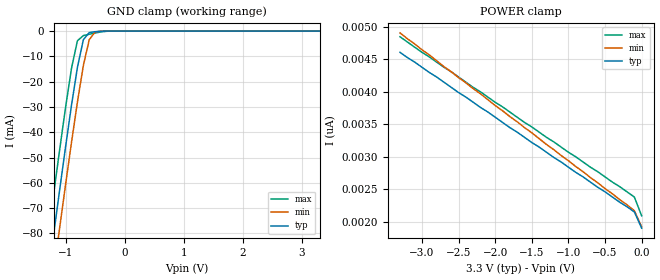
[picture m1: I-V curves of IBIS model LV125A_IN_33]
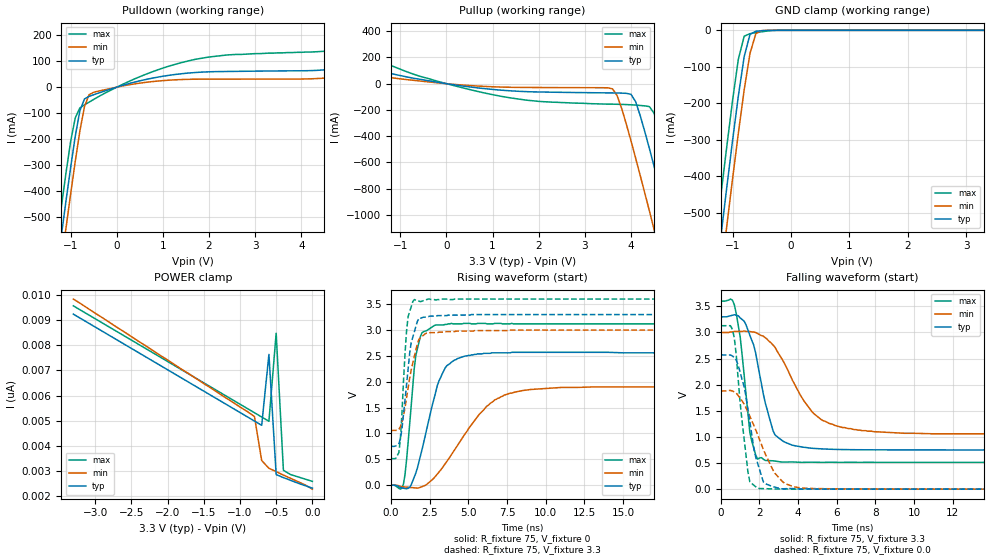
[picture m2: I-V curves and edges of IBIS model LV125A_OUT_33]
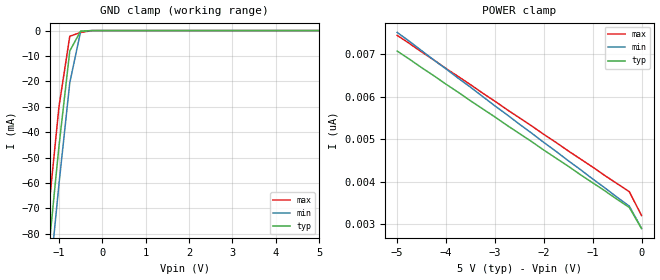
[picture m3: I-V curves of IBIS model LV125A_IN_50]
| TEXAS INSTRUMENTS INCORPORATED
| Standard Linear and Logic Group
| IBIS Model of SN74LV125A
| QUADRUPLE BUS BUFFER GATE WITH 3-STATE OUTPUTS
| SOIC 14-pin (D), SOP 14-pin (NS), SSOP 14-pin (DB), TSSOP 14-pin (PW)
| and TVSOP 14-pin (DGV) Package
[IBIS Ver]   3.2
[Comment Char]  |_char
[File Name]   lv125a.ibs
[File Rev]   2.0 H_die
[Date]   May 26, 2000
[Source]   Data created from HSPICE simulations at TI-SLL.
[Notes]   The following is an IBIS list for the LV125A.
|   Please contact sllibis@ti.com with questions and
|   comments concerning SLL IBIS models.
|   The warning about non-monotonic V-I curves might be reported,
|   but it is nano ampere region and negligible.
[Disclaimer] Property of Texas Instruments Incorporated.  Unauthorized
   reproduction and/or distribution is strictly prohibited.
   This product is protected under copyright law.
   Created 2000, (C) Copyright 2000, Texas Instruments Inc.,
   All Rights Reserved.
   UNLESS THERE IS A SIGNED, WRITTEN AGREEMENT TO THE
   CONTRARY, TEXAS INSTRUMENTS () IS PROVIDING THE IBIS
   MODELS  AND WITHOUT ANY WARRANTY, EXPRESSED OR
   IMPLIED.  TI assumes no liability for:
   1) the accuracy of the IBIS models provided to your
   company;
   2) the proper functioning of these IBIS Models in your
   design or for any resulting applications; or
   3) infringement of patents, copyrights or intellectual
   property rights resulting from your use of these IBIS
   models.
   TI provides IBIS Models as a service to our customers.
   You and your company shall not distribute, sell or give
   these models to anyone else without prior written
   permission from TI.
   TI reserves the right to make changes to our products or
   to discontinue any semiconductor product or service
   without notice, and advises our customers to obtain the
   latest version of relevant information to verify, before
   placing orders, that the information being relied on is
   current.
   Please be aware that your receipt and use of the IBIS
   information provided shall serve as acceptance of these
   terms and conditions.  If you do not accept these terms,
   you should return or destroy the IBIS models and any
   other accompanying information immediately.
|   Component LV125A_D
[Component]   LV125A_D
[Manufacturer]  Texas Instruments, Inc.
[Package]
|   typ   min   max
R_pkg   0.031   0.028   0.034
L_pkg   3.109nH   2.462nH   3.889nH
C_pkg   0.473pF   0.363pF   0.628pF
[Pin]   signal_name   model_name   R_pin   L_pin   C_pin
1   1OE_NOT   LV125A_IN   0.033   3.854nH   0.622pF
2   1A   LV125A_IN   0.032   3.188nH   0.473pF
3   1Y   LV125A_OUT   0.028   2.462nH   0.377pF
4   2OE_NOT   LV125A_IN   0.031   2.596nH   0.363pF
5   2A   LV125A_IN   0.028   2.521nH   0.372pF
6   2Y   LV125A_OUT   0.034   3.250nH   0.476pF
7   GND   GND   0.034   3.889nH   0.628pF
8   3Y   LV125A_OUT   0.034   3.889nH   0.628pF
9   3A   LV125A_IN   0.034   3.250nH   0.476pF
10   3OE_NOT   LV125A_IN   0.028   2.521nH   0.372pF
11   4Y   LV125A_OUT   0.031   2.596nH   0.364pF
12   4A   LV125A_IN   0.028   2.462nH   0.377pF
13   4OE_NOT   LV125A_IN   0.032   3.188nH   0.473pF
14   VCC   POWER   0.033   3.854nH   0.622pF
|   Component LV125A_NS
[Component]   LV125A_NS
[Manufacturer]  Texas Instruments, Inc.
[Package]
|   typ   min   max
R_pkg   0.045   0.039   0.054
L_pkg   3.796nH   2.561nH   4.952nH
C_pkg   0.528pF   0.288pF   0.710pF
[Pin]   signal_name   model_name   R_pin   L_pin   C_pin
1   1OE_NOT   LV125A_IN   0.047   4.867nH   0.706pF
2   1A   LV125A_IN   0.051   4.083nH   0.592pF
3   1Y   LV125A_OUT   0.041   2.915nH   0.376pF
4   2OE_NOT   LV125A_IN   0.039   2.561nH   0.288pF
5   2A   LV125A_IN   0.041   3.101nH   0.430pF
6   2Y   LV125A_OUT   0.047   4.047nH   0.589pF
7   GND   GND   0.051   4.909nH   0.700pF
8   3Y   LV125A_OUT   0.045   4.784nH   0.694pF
9   3A   LV125A_IN   0.054   4.176nH   0.597pF
10   3OE_NOT   LV125A_IN   0.039   3.287nH   0.449pF
11   4Y   LV125A_OUT   0.039   2.586nH   0.294pF
12   4A   LV125A_IN   0.040   2.802nH   0.371pF
13   4OE_NOT   LV125A_IN   0.049   4.080nH   0.593pF
14   VCC   POWER   0.052   4.952nH   0.710pF
|   Component LV125A_DB
[Component]   LV125A_DB
[Manufacturer]  Texas Instruments, Inc.
[Package]
|   typ   min   max
R_pkg   0.044   0.041   0.046
L_pkg   3.551nH   3.258nH   3.927nH
C_pkg   0.402pF   0.360pF   0.421pF
[Pin]   signal_name   model_name   R_pin   L_pin   C_pin
1   1OE_NOT   LV125A_IN   0.046   3.927nH   0.408pF
2   1A   LV125A_IN   0.044   3.587nH   0.421pF
3   1Y   LV125A_OUT   0.041   3.289nH   0.398pF
4   2OE_NOT   LV125A_IN   0.042   3.258nH   0.360pF
5   2A   LV125A_IN   0.041   3.286nH   0.403pF
6   2Y   LV125A_OUT   0.044   3.586nH   0.421pF
7   GND   GND   0.046   3.927nH   0.408pF
8   3Y   LV125A_OUT   0.046   3.927nH   0.408pF
9   3A   LV125A_IN   0.044   3.586nH   0.421pF
10   3OE_NOT   LV125A_IN   0.041   3.286nH   0.403pF
11   4Y   LV125A_OUT   0.043   3.258nH   0.360pF
12   4A   LV125A_IN   0.041   3.289nH   0.398pF
13   4OE_NOT   LV125A_IN   0.044   3.587nH   0.421pF
14   VCC   POWER   0.046   3.927nH   0.408pF
|   Component LV125A_PW
[Component]   LV125A_PW
[Manufacturer]  Texas Instruments, Inc.
[Package]
|   typ   min   max
R_pkg   0.032   0.029   0.035
L_pkg   2.378nH   2.170nH   2.680nH
C_pkg   0.314pF   0.270pF   0.335pF
[Pin]   signal_name   model_name   R_pin   L_pin   C_pin
1   1OE_NOT   LV125A_IN   0.033   2.618nH   0.330pF
2   1A   LV125A_IN   0.031   2.313nH   0.317pF
3   1Y   LV125A_OUT   0.030   2.310nH   0.314pF
4   2OE_NOT   LV125A_IN   0.031   2.173nH   0.272pF
5   2A   LV125A_IN   0.030   2.204nH   0.309pF
6   2Y   LV125A_OUT   0.032   2.315nH   0.317pF
7   GND   GND   0.035   2.680nH   0.335pF
8   3Y   LV125A_OUT   0.033   2.640nH   0.333pF
9   3A   LV125A_IN   0.034   2.347nH   0.319pF
10   3OE_NOT   LV125A_IN   0.029   2.277nH   0.313pF
11   4Y   LV125A_OUT   0.031   2.170nH   0.270pF
12   4A   LV125A_IN   0.031   2.244nH   0.311pF
13   4OE_NOT   LV125A_IN   0.033   2.343nH   0.321pF
14   VCC   POWER   0.035   2.657nH   0.332pF
|   Component LV125A_DGV
[Component]   LV125A_DGV
[Manufacturer]  Texas Instruments, Inc.
[Package]
|   typ   min   max
R_pkg   0.035   0.020   0.045
L_pkg   2.499nH   2.077nH   2.966nH
C_pkg   0.361pF   0.305pF   0.416pF
[Pin]   signal_name   model_name   R_pin   L_pin   C_pin
1   1OE_NOT   LV125A_IN   0.027   2.717nH   0.373pF
2   1A   LV125A_IN   0.037   2.434nH   0.398pF
3   1Y   LV125A_OUT   0.034   2.200nH   0.316pF
4   2OE_NOT   LV125A_IN   0.020   2.077nH   0.309pF
5   2A   LV125A_IN   0.030   2.147nH   0.305pF
6   2Y   LV125A_OUT   0.042   2.580nH   0.408pF
7   GND   GND   0.039   2.921nH   0.385pF
8   3Y   LV125A_OUT   0.033   2.841nH   0.380pF
9   3A   LV125A_IN   0.042   2.611nH   0.410pF
10   3OE_NOT   LV125A_IN   0.038   2.331nH   0.329pF
11   4Y   LV125A_OUT   0.026   2.223nH   0.319pF
12   4A   LV125A_IN   0.034   2.259nH   0.313pF
13   4OE_NOT   LV125A_IN   0.045   2.681nH   0.416pF
14   VCC   POWER   0.042   2.966nH   0.386pF
[Model Selector]   LV125A_IN
LV125A_IN_33   3.3-V Vcc Input Model
LV125A_IN_50   5.0-V Vcc Input Model
[Model Selector]   LV125A_OUT
LV125A_OUT_33   3.3-V Vcc Output Model
LV125A_OUT_50   5.0-V Vcc Output Model
| Models and submodels in the file (4): LV125A_IN_33 (Input), LV125A_OUT_33 (3-state), LV125A_IN_50 (Input), LV125A_OUT_50 (3-state)
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|   Model LV125A_IN_33
[Model]   LV125A_IN_33
Model_type  Input
Polarity   Inverting
Vinl = 0.99
Vinh = 2.31
| variable   typ   min   max
C_comp   1.24pf   0.94pf   1.54pf
[Temperature Range]   25   85   -40
[Voltage Range]   3.3   3.0   3.6
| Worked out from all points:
|   GND clamp passes 1 mA (typ) near -0.61 V on its own axis
[GND Clamp]
|   Voltage   I(typ)   I(min)   I(max)
-3.3V     -460mA     -475mA     -445mA
-1.3V     -97.5mA    -113mA     -81.5mA
-1.2V     -79.9mA    -95mA      -63.9mA
-1.1V     -62.6mA    -77.6mA    -46.7mA
-1V       -45.6mA    -60.5mA    -30mA
-900mV    -29.2mA    -43.9mA    -14.6mA
-800mV    -14.3mA    -28mA      -3.81mA
-700mV    -3.42mA    -13.6mA    -1.78mA
-600mV    -581uA     -3.4mA     -1.25mA
-500mV    -233uA     -353uA     -759uA
-400mV    -58.1uA    -21.9uA    -324uA
3.3V      1.9nA      2.34nA     1.69nA
[POWER Clamp]
|   Voltage   I(typ)   I(min)   I(max)
-3.3V     4.61nA     4.91nA     4.85nA
-3V       4.38nA     4.65nA     4.61nA
-100mV    2.15nA     2.17nA     2.38nA
0V        1.9nA      1.92nA     2.09nA
|   Model LV125A_OUT_33
[Model]   LV125A_OUT_33
Model_type  3-state
Polarity   Non-Inverting
Enable   Active-Low
Vmeas = 1.65v
Cref = 15pf
| variable   typ   min   max
C_comp   6.5pf   4.87pf   8.13pf
[Temperature Range]   25   85   -40
[Voltage Range]   3.3   3.0   3.6
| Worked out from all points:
|   slope of the pulldown table from 0 to 0.495 V, typ, clamps not added: 20.5 ohm
|   slope of the pullup table from 0 to 0.495 V, typ, clamps not added: 20.4 ohm
|   GND clamp passes 1 mA (typ) near -0.48 V on its own axis
|   rising waveform, R_fixture 75, V_fixture 0: 20-80 % time 1.3ns typ, 2.75ns min, 555ps max; typ from 0 V to 2.56 V
|   falling waveform, R_fixture 75, V_fixture 3.3: 20-80 % time 926ps typ, 1.84ns min, 518ps max; typ from 3.3 V to 0.75 V
|   rising waveform, R_fixture 75, V_fixture 3.3: 20-80 % time 569ps typ, 738ps min, 350ps max; typ from 0.75 V to 3.3 V
|   falling waveform, R_fixture 75, V_fixture 0.0: 20-80 % time 755ps typ, 1.31ns min, 498ps max; typ from 2.57 V to 0 V
[Pulldown]
|   Voltage   I(typ)   I(min)   I(max)
-3.3V     -3.5A      -3.6A      -3.4A
-1.3V     -703mA     -808mA     -593mA
-1.2V     -569mA     -674mA     -459mA
-1.1V     -437mA     -541mA     -329mA
-900mV    -189mA     -286mA     -118mA
-800mV    -91.1mA    -169mA     -79.8mA
-700mV    -45.3mA    -74.8mA    -67.8mA
-600mV    -35.4mA    -28.9mA    -57.6mA
-500mV    -29.1mA    -19.5mA    -47.1mA
1.7V      56.3mA     30.7mA     107mA
4.7V      70.2mA     37.1mA     142mA
6.6V      121mA      68.6mA     227mA
[Pullup]
|   Voltage   I(typ)   I(min)   I(max)
-3.3V     228mA      127mA      422mA
-700mV    40.5mA     25.1mA     70.7mA
600mV     -28.8mA    -16.4mA    -52.8mA
3.6V      -70.5mA    -39.4mA    -156mA
3.8V      -72.1mA    -191mA     -158mA
4V        -80.8mA    -435mA     -161mA
4.1V      -137mA     -566mA     -163mA
4.5V      -628mA     -1.11A     -225mA
4.8V      -1.04A     -1.52A     -594mA
5.1V      -1.45A     -1.94A     -1A
5.2V      -1.59A     -2.08A     -1.14A
6.6V      -3.56A     -4.05A     -3.11A
[GND Clamp]
|   Voltage   I(typ)   I(min)   I(max)
-3.3V     -3.5A      -3.6A      -3.39A
-1.3V     -701mA     -807mA     -588mA
-1.2V     -566mA     -672mA     -453mA
-1.1V     -433mA     -539mA     -321mA
-1V       -303mA     -408mA     -193mA
-900mV    -180mA     -282mA     -79.1mA
-800mV    -72mA      -163mA     -16.1mA
-700mV    -10.9mA    -62.8mA    -9.07mA
-600mV    -2.49mA    -8.97mA    -6.42mA
-500mV    -1.18mA    -669uA     -3.99mA
-200mV    -3.04nA    -62.4nA    -8.64uA
3.3V      2.32nA     2.71nA     2.31nA
[POWER Clamp]
|   Voltage   I(typ)   I(min)   I(max)
-3.3V     9.24nA     9.84nA     9.57nA
-800mV    4.99nA     5.17nA     5.32nA
-700mV    4.82nA     3.42nA     5.15nA
-600mV    7.64nA     3.11nA     4.98nA
-500mV    2.86nA     2.98nA     8.48nA
-400mV    2.74nA     2.84nA     3.03nA
-300mV    2.63nA     2.71nA     2.86nA
-100mV    2.42nA     2.45nA     2.68nA
0V        2.32nA     2.28nA     2.59nA
[Ramp]
| variable   typ   min   max
dV/dt_r   1.54E+00/1.29E-09   1.15E+00/2.78E-09   1.88E+00/5.30E-10
dV/dt_f   1.55E+00/8.82E-10   1.18E+00/1.82E-09   1.88E+00/5.32E-10
R_load = 75
[Rising Waveform]
R_fixture = 75
V_fixture = 0
|   Time   V(typ)   V(min)   V(max)
0s        0V         0V         0V
800ps     -59.7mV    -32.6mV    27.2mV
1.6ns     236mV      -54.3mV    2.51V
2ns       690mV      -28.7mV    2.95V
2.8ns     1.7V       147mV      3.09V
3.5ns     2.27V      416mV      3.11V
4.1ns     2.42V      681mV      3.12V
6.1ns     2.55V      1.5V       3.13V
7.7ns     2.56V      1.78V      3.12V
25ns      2.56V      1.9V       3.12V
[Falling Waveform]
R_fixture = 75
V_fixture = 3.3
V_fixture_min = 3.0
V_fixture_max = 3.6
|   Time   V(typ)   V(min)   V(max)
0s        3.3V       3V         3.6V
700ps     3.34V      3.02V      3.53V
1ns       3.28V      3.02V      2.92V
1.5ns     2.95V      3.02V      1.09V
1.9ns     2.41V      2.98V      576mV
2.7ns     1.12V      2.76V      543mV
3.8ns     834mV      2.02V      520mV
5.2ns     772mV      1.33V      513mV
7.3ns     755mV      1.12V      513mV
25ns      750mV      1.06V      512mV
[Rising Waveform]
R_fixture = 75
V_fixture = 3.3
V_fixture_min = 3.0
V_fixture_max = 3.6
|   Time   V(typ)   V(min)   V(max)
0s        750mV      1.05V      512mV
500ps     802mV      1.08V      628mV
600ps     900mV      1.13V      894mV
1ns       1.95V      1.69V      2.99V
1.1ns     2.25V      1.88V      3.26V
1.3ns     2.76V      2.23V      3.45V
1.5ns     2.96V      2.49V      3.59V
1.8ns     3.23V      2.82V      3.56V
2.5ns     3.27V      2.95V      3.6V
25ns      3.3V       3V         3.6V
[Falling Waveform]
R_fixture = 75
V_fixture = 0.0
|   Time   V(typ)   V(min)   V(max)
0s        2.57V      1.88V      3.13V
600ps     2.55V      1.88V      3.06V
900ps     2.37V      1.79V      2.1V
1.4ns     1.53V      1.48V      339mV
1.7ns     804mV      1.23V      78.1mV
2ns       380mV      951mV      12.4mV
2.2ns     139mV      761mV      10.6mV
2.8ns     38.8mV     304mV      2.74mV
4.2ns     3.16mV     22.1mV     2.5mV
25ns      79.9uV     90.5uV     57.2uV
|   Model LV125A_IN_50
[Model]   LV125A_IN_50
Model_type  Input
Polarity   Inverting
Vinl = 1.5
Vinh = 3.5
| variable   typ   min   max
C_comp   1.24pf   0.94pf   1.54pf
[Temperature Range]   25   85   -40
[Voltage Range]   5.0   4.5   5.5
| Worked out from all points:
|   GND clamp passes 1 mA (typ) near -0.52 V on its own axis
[GND Clamp]
|   Voltage   I(typ)   I(min)   I(max)
-5V       -773mA     -786mA     -758mA
-1.5V     -133mA     -148mA     -117mA
-1.25V    -88.7mA    -104mA     -72.7mA
-1V       -45.6mA    -60.5mA    -30mA
-750mV    -7.99mA    -20.5mA    -2.23mA
-500mV    -233uA     -353uA     -759uA
-250mV    -2.63nA    -182nA     -26.9uA
5V        2.9nA      3.64nA     2.54nA
[POWER Clamp]
|   Voltage   I(typ)   I(min)   I(max)
-5V       7.08nA     7.52nA     7.45nA
-1.5V     4.37nA     4.5nA      4.73nA
-250mV    3.4nA      3.43nA     3.77nA
0V        2.9nA      2.91nA     3.21nA
